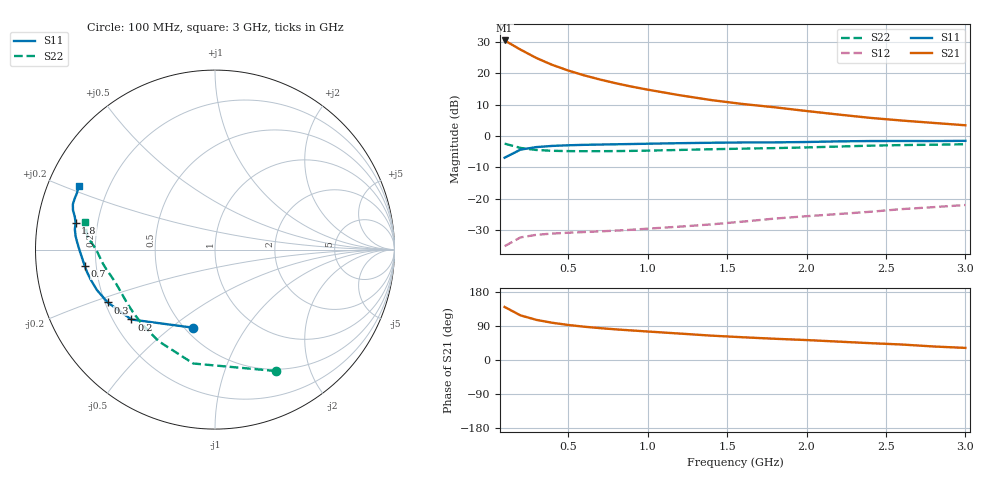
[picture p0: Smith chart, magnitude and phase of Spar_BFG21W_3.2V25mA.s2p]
! Filename: 3_225bfg21.001
! Title: BFG21W
! Bias: Vce=3.2V; Ic=25mA
! Company: NXP Semiconductors NL
! User: Quality&Reliability T&D
! Measure time: 10 Nov 1999 / 11:42:14
#  MHz  S  MA  R 50
! Freq  S11  S21  S12  S22  :
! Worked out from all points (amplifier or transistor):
!   20 points, 100 MHz to 3 GHz, reference 50 ohm
!   highest |S21| = 30.4 dB at 100 MHz (marker M1)
!   |S21| within 3 dB of that: start of sweep to 203.5 MHz
!   unconditionally stable (mu >= 1): 1.137 GHz to end of sweep
!   at 400 MHz: K = 0.47, MSG = 26.8 dB, |S12| = -31.0 dB
!   at 1.2 GHz: K = 1.03, MAG = 19.9 dB, |S12| = -28.8 dB
!   at 3 GHz: K = 1.06, MAG = 11.1 dB, |S12| = -21.9 dB
!   S11 on the Smith chart (normalised r, x): 100 MHz: 0.55, -0.60; 200 MHz: 0.27, -0.34; 300 MHz: 0.21, -0.22; 700 MHz: 0.16, -0.06; 1.8 GHz: 0.12, +0.09; 3 GHz: 0.09, +0.22
100  0.4518 -105.6  32.97 140.0  0.01774 51.3  0.7564 -63.4
200  0.607 -140.1  23.59 117.8  0.02446 37.8  0.646 -100.8
300  0.6665 -153.8  17.36 105.9  0.02688 32.6  0.5994 -121.6
400  0.6955 -161.1  13.49 98.2  0.02816 31.3  0.5817 -134.2
500  0.7117 -166.2  10.99 92.5  0.029 31.6  0.575 -142.5
600  0.7233 -169.8  9.2 87.9  0.02975 32.9  0.5732 -148.3
700  0.7311 -172.7  7.9 84.1  0.03049 35.0  0.5735 -152.7
800  0.7381 -175.2  6.887 80.8  0.03136 37.5  0.5756 -156.3
900  0.7455 -177.4  6.085 78.0  0.03234 40.5  0.5797 -159.3
1000  0.7534 -179.4  5.451 75.2  0.03366 43.1  0.5852 -162.0
1200  0.7684 177.1  4.453 69.8  0.03624 47.9  0.6 -166.4
1400  0.7807 174.4  3.724 64.3  0.03936 52.2  0.6161 -169.9
1600  0.7889 171.8  3.222 60.0  0.0436 56.2  0.6292 -172.9
1800  0.7913 169.0  2.857 56.0  0.0487 59.6  0.6422 -176.0
2000  0.8024 166.8  2.494 52.6  0.05314 62.7  0.6583 -179.3
2200  0.8211 164.5  2.194 48.6  0.0575 64.6  0.6795 177.8
2400  0.8313 162.3  1.942 44.4  0.06246 65.6  0.7017 175.6
2600  0.8319 160.2  1.76 40.9  0.06885 66.1  0.7171 173.5
2800  0.8312 157.7  1.612 35.7  0.07404 65.5  0.7267 171.1
3000  0.8376 155.0  1.48 31.9  0.08006 65.5  0.7391 168.2
